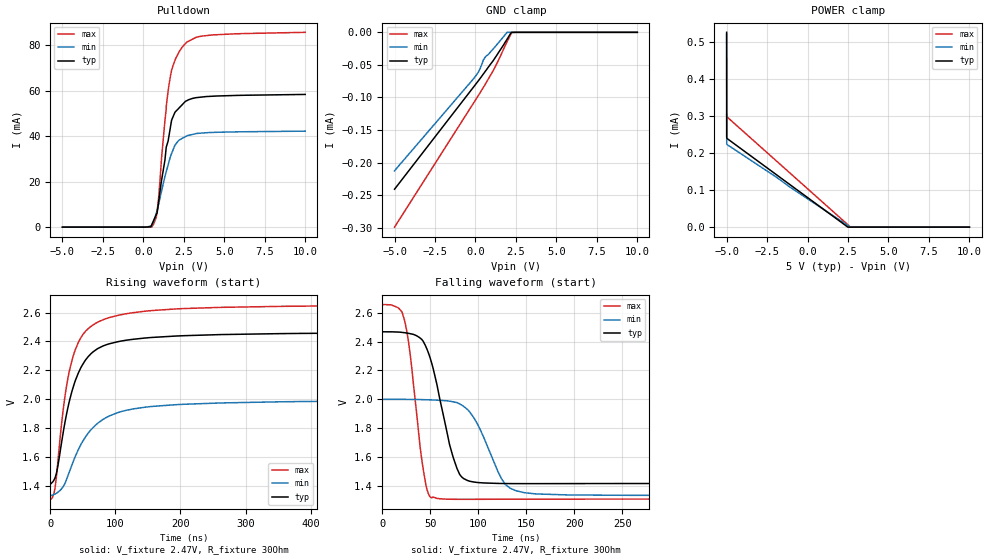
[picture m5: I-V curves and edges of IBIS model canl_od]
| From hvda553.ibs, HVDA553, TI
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|   canl_od Model
[Model]   canl_od
Model_type   I/O_open_drain
Polarity   Non-Inverting
Enable   Active-Low
Vinl = 0.5
Vinh = 0.9
Vmeas = 2.0
Vref = 2.47
Rref = 30
|   typ   min   max
|   (nom PVT)   (fast PVT)   (slow PVT)
C_comp   5.254e-12   4.864e-12   5.945e-12
[Voltage Range]   5   4.68   5.33
[Temperature Range]   27   150   -40
[Pullup Reference]   5   4.68   5.33
[Pulldown Reference]   0   0   0
[Power Clamp Reference]   5   4.68   5.33
[GND Clamp Reference]   0   0   0
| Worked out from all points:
|   slope of the pulldown table from 0 to 0.75 V, typ, clamps not added: 158 ohm
|   falling waveform, V_fixture 2.47V, R_fixture 30Ohm: 20-80 % time 21.5ns typ, 27ns min, 13.7ns max; typ from 2.47 V to 1.41 V
|   rising waveform, V_fixture 2.47V, R_fixture 30Ohm: 20-80 % time 37.2ns typ, 55.9ns min, 30.6ns max; typ from 1.41 V to 2.47 V
[Pulldown]
|   Voltage   I(typ)   I(min)   I(max)
-5V       -413nA     -403.7nA   -492.8nA
511.2mV   956.2uA    613uA      1.891uA
831mV     6.04mA     6.949mA    5.703mA
942.9mV   11.02mA    10.17mA    12.99mA
1.119V    20.29mA    15.66mA    29.88mA
1.332V    29.4mA     22.27mA    46.72mA
1.417V    35.26mA    24.47mA    53.28mA
1.705V    45.34mA    31.67mA    67.7mA
1.955V    50.54mA    36.08mA    73.32mA
2.702V    55.67mA    40.21mA    81.42mA
4.306V    57.58mA    41.65mA    84.53mA
10V       58.35mA    42.21mA    85.66mA
[GND Clamp]
|   Voltage   I(typ)   I(min)   I(max)
-5V       -240.9uA   -212.9uA   -299.2uA
-118.8mV  -84.09uA   -71.33uA   -108.7uA
185.4mV   -74.23uA   -60.99uA   -96.8uA
297.8mV   -70.52uA   -55.08uA   -92.36uA
485mV     -64.17uA   -42.73uA   -84.76uA
575.2mV   -61.08uA   -39.26uA   -81.08uA
1.119V    -42.72uA   -24.89uA   -57.92uA
1.95V     -10.86uA   -73.12nA   -14.56uA
2.233V    -124.1nA   0A         -211.4nA
10.01V    0A         0A         0A
[POWER Clamp]
|   Voltage   I(typ)   I(min)   I(max)
-5.005V   526.7uA    521.2uA    304.3uA
-5V       243.1uA    226uA      302.4uA
-4.967V   239.6uA    222.9uA    297.7uA
2.49V     38.46nA    4.474uA    6.559uA
2.654V    0A         0A         150.2nA
10.01V    0A         0A         0A
[Ramp]
R_load = 30
|   typ   min   max
dV/dt_r   0.631309/3.71274e-08   0.398704/5.58298e-08   0.810149/3.05664e-08
dV/dt_f   0.632559/2.13882e-08   0.399974/2.69363e-08   0.811508/1.37096e-08
[Falling Waveform]
V_fixture = 2.47V
V_fixture_min = 2V
V_fixture_max = 2.66V
R_fixture = 30Ohm
|   Time   V(typ)   V(min)   V(max)
0s        2.469V     1.999V     2.658V
22.8ns    2.463V     1.999V     2.556V
28.8ns    2.456V     1.999V     2.321V
42.2ns    2.406V     1.997V     1.53V
51.2ns    2.255V     1.995V     1.316V
78ns      1.515V     1.976V     1.304V
100.2ns   1.421V     1.814V     1.305V
128ns     1.414V     1.41V      1.305V
160.2ns   1.413V     1.342V     1.306V
1.5us     1.414V     1.332V     1.306V
[Rising Waveform]
V_fixture = 2.47V
V_fixture_min = 2V
V_fixture_max = 2.66V
R_fixture = 30Ohm
|   Time   V(typ)   V(min)   V(max)
0s        1.414V     1.332V     1.306V
7ns       1.451V     1.342V     1.376V
23ns      1.849V     1.421V     2.033V
30ns      1.998V     1.504V     2.209V
38.4ns    2.127V     1.603V     2.342V
49.6ns    2.239V     1.706V     2.445V
65.4ns    2.327V     1.802V     2.514V
108.6ns   2.402V     1.913V     2.585V
354.8ns   2.454V     1.982V     2.643V
1.5us     2.467V     1.997V     2.656V
